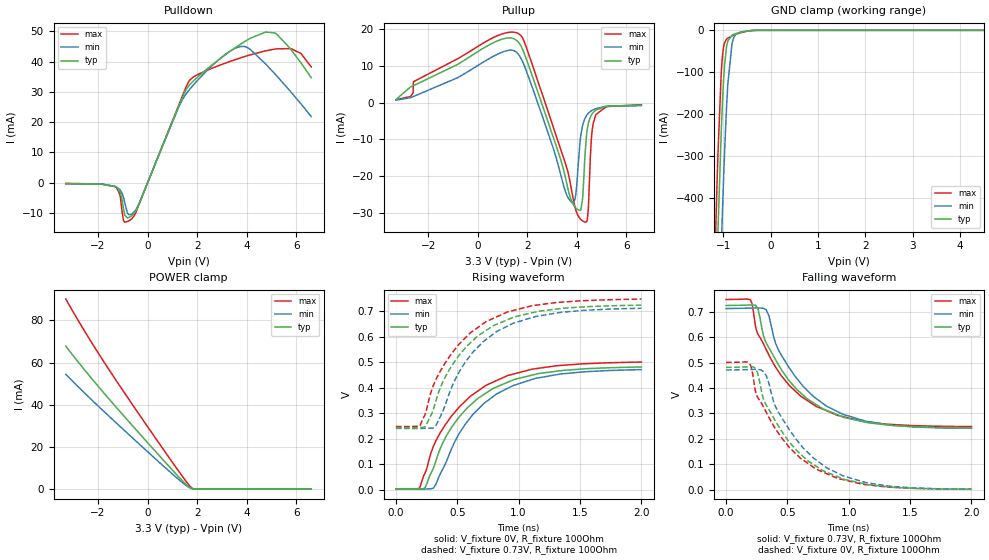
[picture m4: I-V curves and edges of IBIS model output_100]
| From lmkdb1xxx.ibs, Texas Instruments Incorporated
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[Model]   output_100
Model_type   Output
Polarity   Non-Inverting
Vmeas = 0.365
Vref = 0
Cref = 2pF
Rref = 100000
|   typ   min   max
C_comp   5pF   4.5pF   5.5pF
[Voltage Range]   3.3   3.135   3.465
[Temperature Range]   27   125   -40
[Pullup Reference]   3.3   3.135   3.465
[Pulldown Reference]   0   -0   -0
[Power Clamp Reference]   3.3   3.135   3.465
[GND Clamp Reference]   0   0   0
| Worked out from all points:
|   slope of the pulldown table from 0 to 0.495 V, typ, clamps not added: 49.6 ohm
|   GND clamp passes 1 mA (typ) near -0.44 V on its own axis
|   falling waveform, V_fixture 0.73V, R_fixture 100Ohm: 20-80 % time 423ps typ, 419ps min, 432ps max; typ from 0.725 V to 0.244 V
|   rising waveform, V_fixture 0V, R_fixture 100Ohm: 20-80 % time 439ps typ, 430ps min, 448ps max; typ from 0.002 V to 0.482 V
|   rising waveform, V_fixture 0.73V, R_fixture 100Ohm: 20-80 % time 425ps typ, 409ps min, 435ps max; typ from 0.243 V to 0.725 V
|   falling waveform, V_fixture 0V, R_fixture 100Ohm: 20-80 % time 427ps typ, 422ps min, 437ps max; typ from 0.481 V to 0.002 V
[Pulldown]
|   Voltage   I(typ)   I(min)   I(max)
-3.3V     -286.5uA   -353.3uA   -246.3uA
-1.31V    -1.255mA   -1.229mA   -1.291mA
-1.122V   -2.864mA   -2.235mA   -3.846mA
-973.5mV  -8.577mA   -4.786mA   -12.45mA
-815.1mV  -11.64mA   -10.01mA   -12.8mA
-636.9mV  -10.85mA   -10.31mA   -11.87mA
1.68V     32.15mA    30.66mA    33.65mA
3.62V     45.03mA    44.67mA    40.86mA
4.125V    47.59mA    44.08mA    42.16mA
5.135V    49.45mA    35.92mA    44.11mA
6.184V    39.58mA    26.04mA    42.68mA
6.6V      34.67mA    21.84mA    38.22mA
[GND Clamp]
|   Voltage   I(typ)   I(min)   I(max)
-3.3V     -10.93A    -11.17A    -10.79A
-1.211V   -881.9mA   -1.2A      -686.4mA
-1.132V   -556.2mA   -867.4mA   -367.3mA
-1.112V   -480mA     -787.6mA   -296mA
-1.033V   -214.4mA   -487.8mA   -84.32mA
-1.013V   -162.8mA   -419.6mA   -57.31mA
-973.5mV  -84.96mA   -294.9mA   -30.14mA
-904.2mV  -25.65mA   -128.9mA   -18.66mA
-815.1mV  -11.51mA   -31.82mA   -13.47mA
-785.4mV  -9.977mA   -19.98mA   -11.99mA
-320.1mV  -97.64uA   -117.8uA   -83.69uA
6.6V      0A         0A         0A
[Pullup]
|   Voltage   I(typ)   I(min)   I(max)
-3.3V     799.7uA    638.7uA    780.9uA
709.5mV   16.5mA     12.84mA    17.9mA
1.66V     16.22mA    12.94mA    18.65mA
3.759V    -26.33mA   -26.89mA   -22.82mA
3.957V    -28.65mA   -24.89mA   -29.19mA
4.165V    -28.99mA   -8.611mA   -31.82mA
4.234V    -25.87mA   -6.119mA   -32.18mA
4.333V    -13.6mA    -4.19mA    -32.5mA
4.462V    -5.662mA   -2.912mA   -28.8mA
4.6V      -3.186mA   -2.169mA   -8.56mA
4.759V    -2.076mA   -1.67mA    -3.395mA
6.6V      -696.6uA   -862.4uA   -599.2uA
[POWER Clamp]
|   Voltage   I(typ)   I(min)   I(max)
-3.3V     67.84mA    54.47mA    90.13mA
-2.27V    52.65mA    42.51mA    69.74mA
-1.221V   38.23mA    30.93mA    50.7mA
1.175V    6.833mA    5.39mA     9.808mA
1.601V    1.727mA    1.368mA    2.963mA
1.789V    238.8uA    261.3uA    521.2uA
1.977V    4.569uA    9.608uA    7.599uA
6.6V      0A         0A         0A
[Ramp]
R_load = 100
|   typ   min   max
dV/dt_r   0.287957/4.38772e-10   0.281661/4.29919e-10   0.299516/4.47719e-10
dV/dt_f   0.288655/4.23447e-10   0.282751/4.18662e-10   0.300125/4.31928e-10
[Falling Waveform]
V_fixture = 0.73V
V_fixture_min = 0.72V
V_fixture_max = 0.75V
R_fixture = 100Ohm
C_fixture = 0F
|   Time   V(typ)   V(min)   V(max)
0s        724.8mV    712.7mV    748.4mV
197.7ps   727.2mV    714.5mV    747.5mV
258.8ps   714mV      715.1mV    612.7mV
305.5ps   604.8mV    713.5mV    573.4mV
326.8ps   578.4mV    708.2mV    552mV
426.3ps   492.1mV    549.9mV    465.7mV
577.7ps   393.6mV    437mV      381.9mV
734.6ps   334.8mV    358.6mV    327.7mV
1.137ns   265.7mV    269.4mV    267.6mV
2ns       243.7mV    241.5mV    248.2mV
[Rising Waveform]
V_fixture = 0V
V_fixture_min = 0V
V_fixture_max = 0V
R_fixture = 100Ohm
C_fixture = 0F
|   Time   V(typ)   V(min)   V(max)
0s        1.636mV    1.822mV    1.828mV
185.9ps   2.046mV    1.568mV    3.367mV
239.9ps   9.215mV    1.995mV    67.78mV
304.4ps   82.54mV    5.425mV    168.8mV
378.1ps   179.9mV    77.01mV    236mV
454.5ps   245.4mV    161.4mV    289.3mV
563.3ps   311.3mV    255.6mV    346.4mV
734.6ps   379.2mV    344.4mV    409.7mV
1.137ns   452.7mV    436.7mV    474.9mV
2ns       481.6mV    471.3mV    501mV
[Rising Waveform]
V_fixture = 0.73V
V_fixture_min = 0.72V
V_fixture_max = 0.75V
R_fixture = 100Ohm
C_fixture = 0F
|   Time   V(typ)   V(min)   V(max)
0s        242.9mV    240.2mV    247.8mV
197.7ps   244.2mV    240mV      251.9mV
239.9ps   247.6mV    240.6mV    298.9mV
304.4ps   314.3mV    241.4mV    408.2mV
378.1ps   418.7mV    303.6mV    478.8mV
454.5ps   486.3mV    402mV      535mV
563.3ps   555.2mV    499.3mV    595mV
734.6ps   625mV      589.6mV    660mV
1.137ns   697.7mV    680.1mV    724.2mV
2ns       724.7mV    712.4mV    748.5mV
[Falling Waveform]
|Gnd
V_fixture = 0V
V_fixture_min = 0V
V_fixture_max = 0V
R_fixture = 100Ohm
C_fixture = 0F
|   Time   V(typ)   V(min)   V(max)
0s        481.3mV    470.8mV    500.7mV
185.9ps   483.9mV    472.6mV    498.8mV
210.9ps   484mV      473mV      472.3mV
258.8ps   457.6mV    473.1mV    361.5mV
304.4ps   357.4mV    464.6mV    326.4mV
426.3ps   250.5mV    305.3mV    222.4mV
577.7ps   152.5mV    194.5mV    137.1mV
734.6ps   92.04mV    116.4mV    80.64mV
1.137ns   22.13mV    27.89mV    19.85mV
2ns       1.796mV    2.022mV    2.068mV
